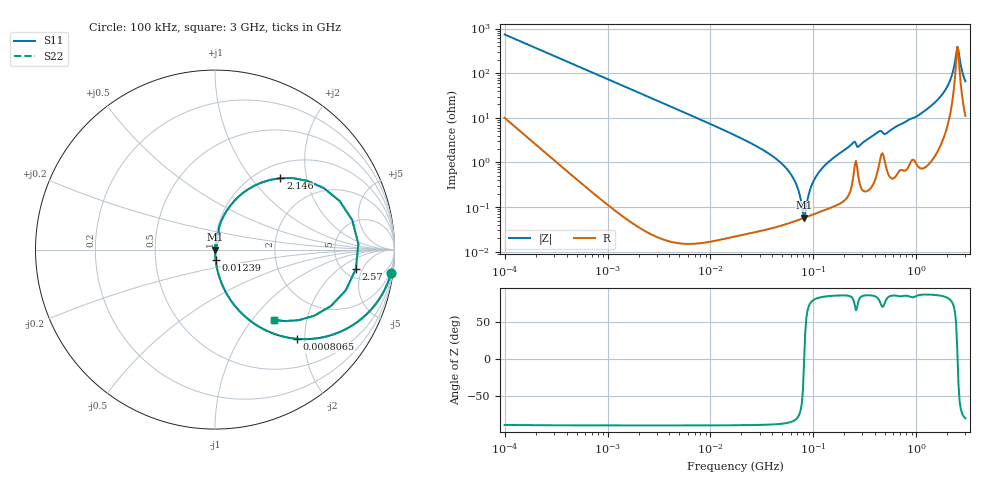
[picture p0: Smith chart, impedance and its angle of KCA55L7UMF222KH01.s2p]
!Murata Part Number: KCA55L7UMF222KH01
!These Parameters are Measured in Series Mode Connection
!Data Generated on Jan 08, 2026
!  o--ll--o
!Port1  Port2
!  o------o
!Operation Temp=25[degC], DC Bias Voltage=0[V]
!Freq. Start=100[kHz] Stop=3[GHz] 401[Steps]
# Hz S RI R 50
!Freq.(Hz) S11(Real) S11(Imag) S21(Real) S21(Imag) S12(Real) S12(Imag) S22(Real) S22(Imag)
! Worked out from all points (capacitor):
!   401 points, 100 kHz to 3 GHz, reference 50 ohm
!   read as one part in series: C = 2.16 nF near 105.3 kHz
!   lowest |Z| = 57.5 mohm at 81.31 MHz (marker M1)
!   series resonance near 81.44 MHz, so ESL is about 1.8 nH
!   S11 on the Smith chart (normalised r, x): 100 kHz: 1, -15; 806.5 kHz: 1.00, -1.83; 12.39 MHz: 1.00, -0.12; 2.146 GHz: 1.26, +1.41; 2.57 GHz: 6.45, -3.72; 3 GHz: 1.22, -1.29
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100000  0.9802 -0.1329  0.0198 0.1329  0.0198 0.1329  0.9802 -0.1329
266273  0.8833 -0.3184  0.1167 0.3184  0.1167 0.3184  0.8833 -0.3184
562235  0.632 -0.481  0.368 0.481  0.368 0.481  0.632 -0.481
806524  0.4554 -0.4971  0.5446 0.4971  0.5446 0.4971  0.4554 -0.4971
3161081  0.0516 -0.2208  0.9484 0.2208  0.9484 0.2208  0.0516 -0.2208
1.238951e7  0.00354 -0.0578  0.9965 0.0578  0.9965 0.0578  0.00354 -0.0578
1.77727e7  0.00177 -0.0393  0.9982 0.0393  0.9982 0.0393  0.00177 -0.0393
5.383243e7  0.000471 -0.00765  0.9995 0.00765  0.9995 0.00765  0.000471 -0.00765
6.788584e7  0.000504 -0.00328  0.9995 0.00328  0.9995 0.00328  0.000504 -0.00328
8.130716e7  0.000574 -2.99e-05  0.9994 2.99e-05  0.9994 2.99e-05  0.000574 -2.99e-05
9.738194e7  0.000681 0.00321  0.9993 -0.00321  0.9993 -0.00321  0.000681 0.00321
1.293002e8  0.000932 0.00855  0.9991 -0.00855  0.9991 -0.00855  0.000932 0.00855
2.400085e8  0.00432 0.0262  0.9957 -0.0262  0.9957 -0.0262  0.00432 0.0262
2.801453e8  0.00409 0.0232  0.9959 -0.0232  0.9959 -0.0232  0.00409 0.0232
4.231245e8  0.00883 0.0465  0.9912 -0.0465  0.9912 -0.0465  0.00883 0.0465
5.475153e8  0.00733 0.0495  0.9927 -0.0495  0.9927 -0.0495  0.00733 0.0495
1.575075e9  0.0678 0.2202  0.9322 -0.2202  0.9322 -0.2202  0.0678 0.2202
2.145926e9  0.3641 0.3979  0.6359 -0.3979  0.6359 -0.3979  0.3641 0.3979
2.318426e9  0.6062 0.3427  0.3938 -0.3427  0.3938 -0.3427  0.6062 0.3427
2.570185e9  0.785 -0.1073  0.215 0.1073  0.215 0.1073  0.785 -0.1073
2.776789e9  0.5536 -0.3681  0.4464 0.3681  0.4464 0.3681  0.5536 -0.3681
3e9  0.3272 -0.3917  0.6728 0.3917  0.6728 0.3917  0.3272 -0.3917
